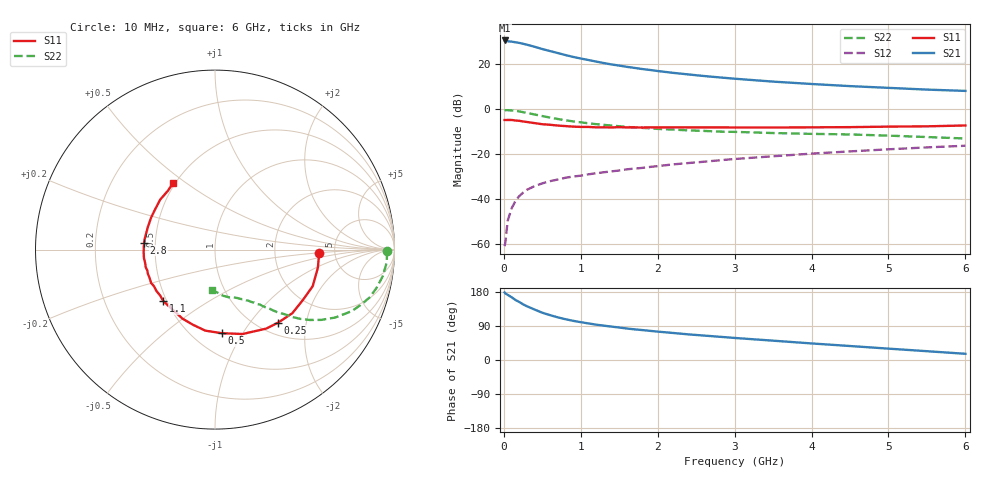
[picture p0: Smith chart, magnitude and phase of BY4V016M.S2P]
! SIEMENS Small Signal Semiconductors
! BFY420
! Si NPN RF SIEGET Grounded Emitter Transistor in MICRO-X
! VCE = 4 V  IC = 16 mA
! Common Emitter S-Parameters:  October  1996
# GHz  S  MA  R  50
!  f  S11  S21  S12  S22
! GHz  MAG  ANG  MAG  ANG  MAG  ANG  MAG  ANG
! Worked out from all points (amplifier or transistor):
!   36 points, 10 MHz to 6 GHz, reference 50 ohm
!   highest |S21| = 30.7 dB at 10 MHz (marker M1)
!   |S21| within 3 dB of that: start of sweep to 418.4 MHz
!   unconditionally stable (mu >= 1): start of sweep to 21.03 MHz; 2.202 GHz to end of sweep
!   at 250 MHz: K = 0.31, MSG = 33.2 dB, |S12| = -37.1 dB
!   at 1.4 GHz: K = 0.86, MSG = 23.8 dB, |S12| = -27.6 dB
!   at 6 GHz: K = 1.07, MAG = 10.7 dB, |S12| = -16.2 dB
!   S11 on the Smith chart (normalised r, x): 10 MHz: 3.75, -0.22; 250 MHz: 1.21, -1.39; 500 MHz: 0.68, -0.81; 1.1 GHz: 0.48, -0.33; 2.8 GHz: 0.43, +0.04; 6 GHz: 0.49, +0.45
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0.01  0.5803 -1.9  34.27 178.3  0.0009 34.3  0.9585 -0.5
0.02  0.5802 -3.7  33.99 175.7  0.0011 55.1  0.958 -1.4
0.05  0.582 -10.0  32.86 171.9  0.0033 74.0  0.9598 -4.2
0.1  0.5813 -20.5  32.31 165.9  0.0062 76.6  0.9464 -9.0
0.15  0.5647 -29.7  31.23 158.5  0.0091 71.3  0.9251 -13.3
0.2  0.5577 -39.5  30.25 153.2  0.0117 71.7  0.9022 -17.2
0.25  0.5379 -49.1  28.93 147.0  0.014 66.5  0.8677 -20.8
0.3  0.5244 -57.1  27.58 141.8  0.0162 66.2  0.8373 -24.1
0.4  0.4947 -71.9  24.79 133.1  0.0196 62.7  0.7704 -29.4
0.5  0.4673 -85.4  22.07 124.7  0.0225 60.4  0.7096 -33.5
0.7  0.4362 -106.5  18 112.6  0.0274 57.7  0.6117 -39.1
0.8  0.425 -115.3  16.22 107.7  0.03 55.9  0.5728 -41.0
0.9  0.4134 -121.6  14.75 103.4  0.032 56.1  0.5406 -42.3
1.1  0.4067 -135.0  12.56 96.5  0.0358 56.4  0.4905 -45.2
1.3  0.3994 -144.7  10.76 90.6  0.0398 56.2  0.4514 -47.1
1.6  0.397 -157.1  8.85 83.0  0.0463 56.0  0.4071 -50.1
2.2  0.3987 -173.4  6.51 71.3  0.0596 55.6  0.3554 -55.2
2.8  0.397 174.4  5.16 61.4  0.0735 53.5  0.32 -59.9
3.5  0.3947 161.6  4.155 51.0  0.0904 50.0  0.2974 -65.2
4.5  0.4026 145.3  3.297 36.9  0.116 43.0  0.2766 -73.9
5.5  0.4195 129.0  2.759 23.2  0.1425 34.7  0.2422 -85.9
6  0.4384 121.9  2.58 16.4  0.155 30.1  0.2248 -93.8
